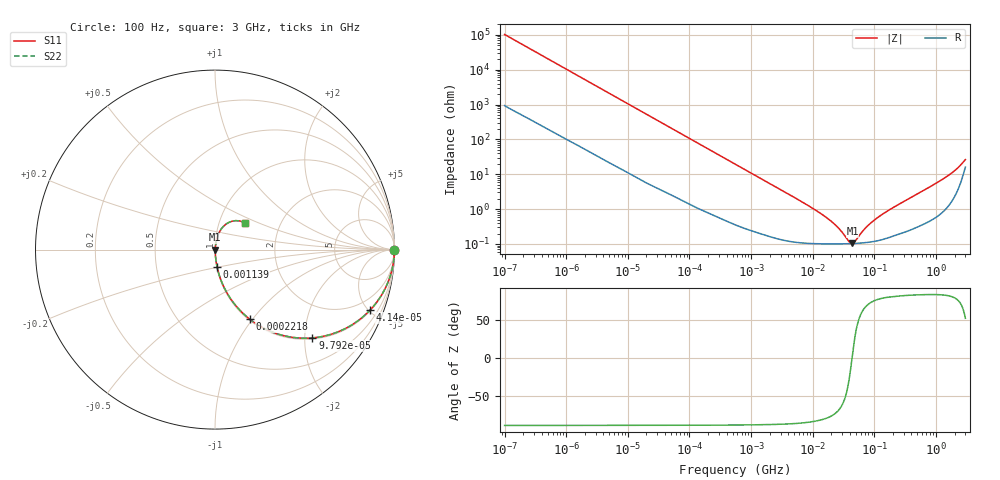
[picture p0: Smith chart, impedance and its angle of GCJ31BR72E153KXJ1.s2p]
!Murata Part Number: GCJ31BR72E153KXJ1
!These Parameters are Measured in Series Mode Connection
!Data Generated on Mar 13, 2026
!  o--ll--o
!Port1  Port2
!  o------o
!Operation Temp=25[degC], DC Bias Voltage=0[V]
!Freq. Start=100[Hz] Stop=3[GHz] 401[Steps]
# Hz S RI R 50
!Freq.(Hz) S11(Real) S11(Imag) S21(Real) S21(Imag) S12(Real) S12(Imag) S22(Real) S22(Imag)
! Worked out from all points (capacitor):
!   401 points, 100 Hz to 3 GHz, reference 50 ohm
!   read as one part in series: C = 15.6 nF near 109 Hz
!   lowest |Z| = 103 mohm at 44.18 MHz (marker M1)
!   series resonance near 43.41 MHz, so ESL is about 860 pH
!   S11 on the Smith chart (normalised r, x): 100 Hz: open; 41.4 kHz: 1.06, -5.13; 97.92 kHz: 1.03, -2.18; 221.8 kHz: 1.01, -0.97; 1.139 MHz: 1.00, -0.19; 3 GHz: 1.32, +0.42
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100  1 -0.000979  9.9e-06 0.000979  9.9e-06 0.000979  1 -0.000979
1788  0.9995 -0.0172  0.000468 0.0172  0.000468 0.0172  0.9995 -0.0172
9582  0.9908 -0.0902  0.00917 0.0902  0.00917 0.0902  0.9908 -0.0902
31977  0.9139 -0.2749  0.0861 0.2749  0.0861 0.2749  0.9139 -0.2749
41399  0.865 -0.3359  0.135 0.3359  0.135 0.3359  0.865 -0.3359
60986  0.7502 -0.4268  0.2498 0.4268  0.2498 0.4268  0.7502 -0.4268
97915  0.5429 -0.4918  0.4571 0.4918  0.4571 0.4918  0.5429 -0.4918
144239  0.3573 -0.4725  0.6427 0.4725  0.6427 0.4725  0.3573 -0.4725
221826  0.1938 -0.3879  0.8062 0.3879  0.8062 0.3879  0.1938 -0.3879
547723  0.0408 -0.1891  0.9592 0.1891  0.9592 0.1891  0.0408 -0.1891
1138514  0.0113 -0.0945  0.9887 0.0945  0.9887 0.0945  0.0113 -0.0945
9794414  0.00114 -0.0107  0.9989 0.0107  0.9989 0.0107  0.00114 -0.0107
2.12544e7  0.00102 -0.00395  0.999 0.00395  0.999 0.00395  0.00102 -0.00395
2.751729e7  0.00101 -0.0024  0.999 0.0024  0.999 0.0024  0.00101 -0.0024
3.882828e7  0.00102 -0.000567  0.999 0.000567  0.999 0.000567  0.00102 -0.000567
4.418008e7  0.00103 9e-05  0.999 -9e-05  0.999 -9e-05  0.00103 9e-05
4.815176e7  0.00104 0.000528  0.999 -0.000528  0.999 -0.000528  0.00104 0.000528
8.425944e7  0.00114 0.0036  0.9989 -0.0036  0.9989 -0.0036  0.00114 0.0036
1.751444e8  0.00163 0.0094  0.9984 -0.0094  0.9984 -0.0094  0.00163 0.0094
1.642185e9  0.0218 0.0925  0.9782 -0.0925  0.9782 -0.0925  0.0218 0.0925
2.317205e9  0.0584 0.1396  0.9416 -0.1396  0.9416 -0.1396  0.0584 0.1396
3e9  0.1647 0.1501  0.8353 -0.1501  0.8353 -0.1501  0.1647 0.1501
